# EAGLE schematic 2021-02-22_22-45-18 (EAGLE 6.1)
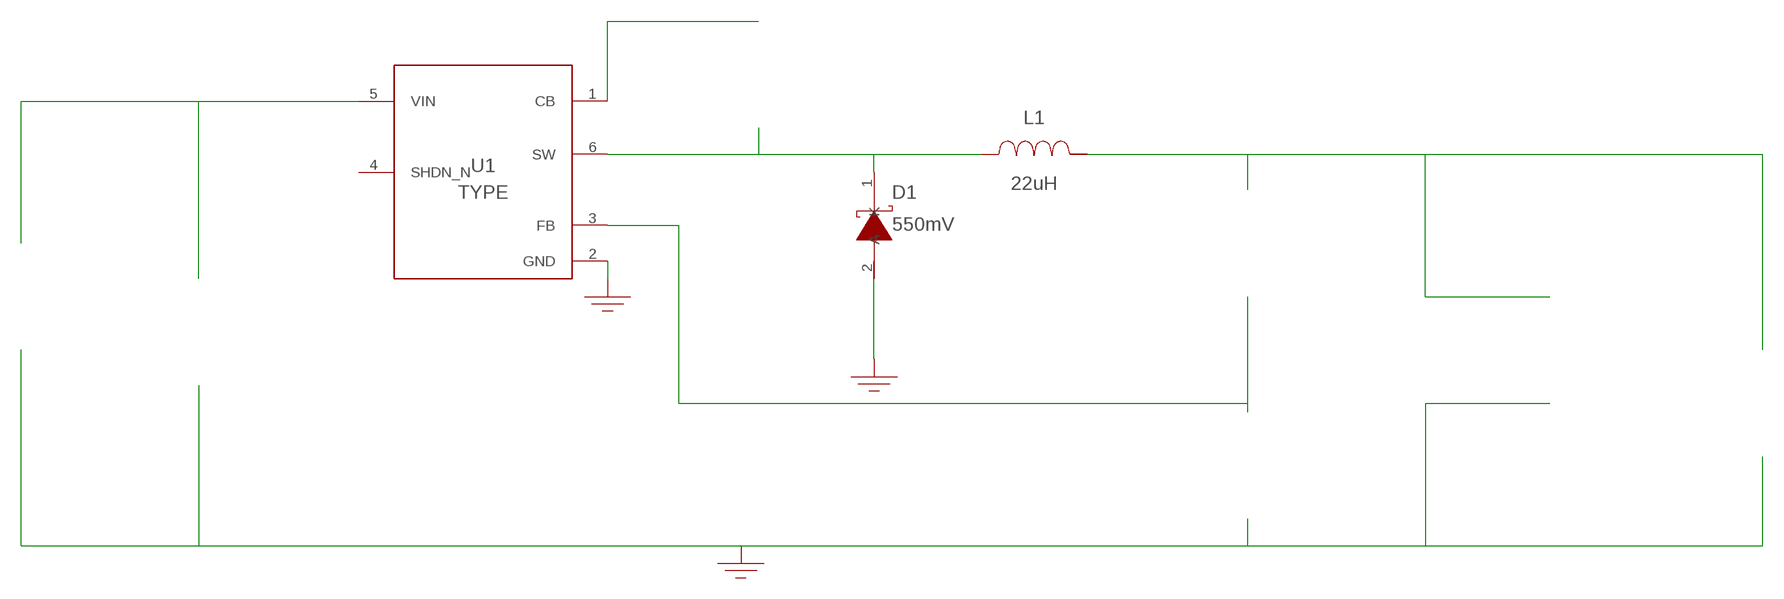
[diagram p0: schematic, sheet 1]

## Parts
CBOOT  100nF  C0805C104M5RACTUC0805C104M5RACTU  [0805]  (not placed on a sheet)
CIN  4.7uF  GRM31CR71H475KA12LGRM31CR71H475KA12L  [1206]  (not placed on a sheet)
COUT  10uF  C3216X6S1V106K160ACC3216X6S1V106K160AC  [1206_180]  (not placed on a sheet)
COUT_2  10uF  C3216X6S1V106K160ACC3216X6S1V106K160AC  [1206_180]  (not placed on a sheet)
D1  550mV  SS24FLSS24FL  [SOD-123F]
GND  WB_GND  WB_GNDWB_GND  [WB_GND]
GND2  WB_GND  WB_GNDWB_GND  [WB_GND]
GND4  WB_GND  WB_GNDWB_GND  [WB_GND]
IOUT  WB_CURRENT_LOAD  WB_CURRENT_LOADWB_CURRENT_LOAD  [WB_CURRENT_LOAD]  (not placed on a sheet)
L1  22uH  NPI105C220MTRFNPI105C220MTRF  [IND_NPI105C]
RFBB  20k  CRCW040220K0FKEDCRCW040220K0FKED  [0402]  (not placed on a sheet)
RFBT  111k  RT0805BRD07111KLRT0805BRD07111KL  [0805]  (not placed on a sheet)
U1  LMR14010ADDCR  LMR14010ADDCRLMR14010ADDCR  [DDC0006A_N]
VIN  WB_BATTERY  WB_BATTERYWB_BATTERY  [WB_BATTERY]  (not placed on a sheet)

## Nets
0: Cin.2@2 Cout.2@2 Cout_2.2@2 D1.2(A) GND2.1 GND4.1 GND.1 Iout.-@2 Rfbb.2@2 U1.2(GND) Vin.-@2
1: Cboot.1@1 U1.1(CB)
2: Rfbb.1@1 Rfbt.2@2 U1.3(FB)
4: Cin.1@1 U1.5(VIN) Vin.+@1
5: Cout.1@1 Cout_2.1@1 Iout.+@1 L1.2 Rfbt.1@1
6: Cboot.2@2 D1.1(K) L1.1 U1.6(SW)
Unconnected: CBOOT.1 CBOOT.2 CIN.1 CIN.2 COUT.1 COUT.2 COUT_2.1 COUT_2.2 IOUT.1(+) IOUT.2(-) RFBB.1 RFBB.2 RFBT.1 RFBT.2 U1.4(SHDN_N) VIN.1(+) VIN.2(-)

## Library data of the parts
CBOOT = AcceleratedDesigns_Lib:C0805C104M5RACTU; Cap: 1.0E-7; ESR: 0.064; IRMS: 1.64; Manufacturer_Name: Kemet; Manufacturer_Part_Number: C0805C104M5RACTU; VDC: 50.0; Vendor: Kemet
CIN = AcceleratedDesigns_Lib:GRM31CR71H475KA12L; Cap: 4.7E-6; ESR: 0.0; IRMS: 0.0; Manufacturer_Name: MuRata; Manufacturer_Part_Number: GRM31CR71H475KA12L; VDC: 50.0; Vendor: MuRata
COUT COUT_2 = AcceleratedDesigns_Lib:C3216X6S1V106K160AC; Cap: 1.0E-5; Datasheet_URL: https://product.tdk.com/en/search/capacitor/ceramic/mlcc/info?part%5Fno%3DC3216X6S1V106K160AC; ESR: 0.002229; IRMS: 4.85932; Manufacturer_Name: TDK; Manufacturer_Part_Number: C3216X6S1V106K160AC; VDC: 35.0; Vendor: TDK
D1 = AcceleratedDesigns_Lib:SS24FL; Datasheet_URL: https://www.fairchildsemi.com/datasheets/SS/SS24FL.pdf; Io: 2.0; Manufacturer_Name: Fairchild Semiconductor; Manufacturer_Part_Number: SS24FL; VFatIo: 0.55; VRRM: 40.0; Vendor: Fairchild Semiconductor
GND GND2 GND4 = AcceleratedDesigns_Lib:WB_GND; Manufacturer_Name: WB_GND; Manufacturer_Part_Number: WB_GND; PowerPortType: POWER_GROUND; Value: Value
IOUT = AcceleratedDesigns_Lib:WB_CURRENT_LOAD; Manufacturer_Name: WB_CURRENT_LOAD; Manufacturer_Part_Number: WB_CURRENT_LOAD; PowerPortType: POWER_GROUND; Value: Value
L1 = AcceleratedDesigns_Lib:NPI105C220MTRF; DCR: 0.1; IDC: 1.95; L: 2.2E-5; Manufacturer_Name: NIC Components; Manufacturer_Part_Number: NPI105C220MTRF; Vendor: NIC Components
RFBB = AcceleratedDesigns_Lib:CRCW040220K0FKED; Manufacturer_Name: Vishay-Dale; Manufacturer_Part_Number: CRCW040220K0FKED; Power: 0.063; Resistance: 20000.0; Tolerance: 1.0; Vendor: Vishay-Dale
RFBT = AcceleratedDesigns_Lib:RT0805BRD07111KL; Manufacturer_Name: Yageo; Manufacturer_Part_Number: RT0805BRD07111KL; Power: 0.125; Resistance: 111000.0; Tolerance: 0.1; Vendor: Yageo America
U1 = AcceleratedDesigns_Lib:LMR14010ADDCR; Manufacturer: Texas Instruments; Manufacturer_Name: Texas Instruments; Manufacturer_Part_Number: LMR14010ADDCR; PartNumber: LMR14010ADDCR; RefDes: RefDes; TYPE: TYPE; Value: Value
VIN = AcceleratedDesigns_Lib:WB_BATTERY; Manufacturer_Name: WB_BATTERY; Manufacturer_Part_Number: WB_BATTERY; PowerPortType: POWER_GROUND; Value: Value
